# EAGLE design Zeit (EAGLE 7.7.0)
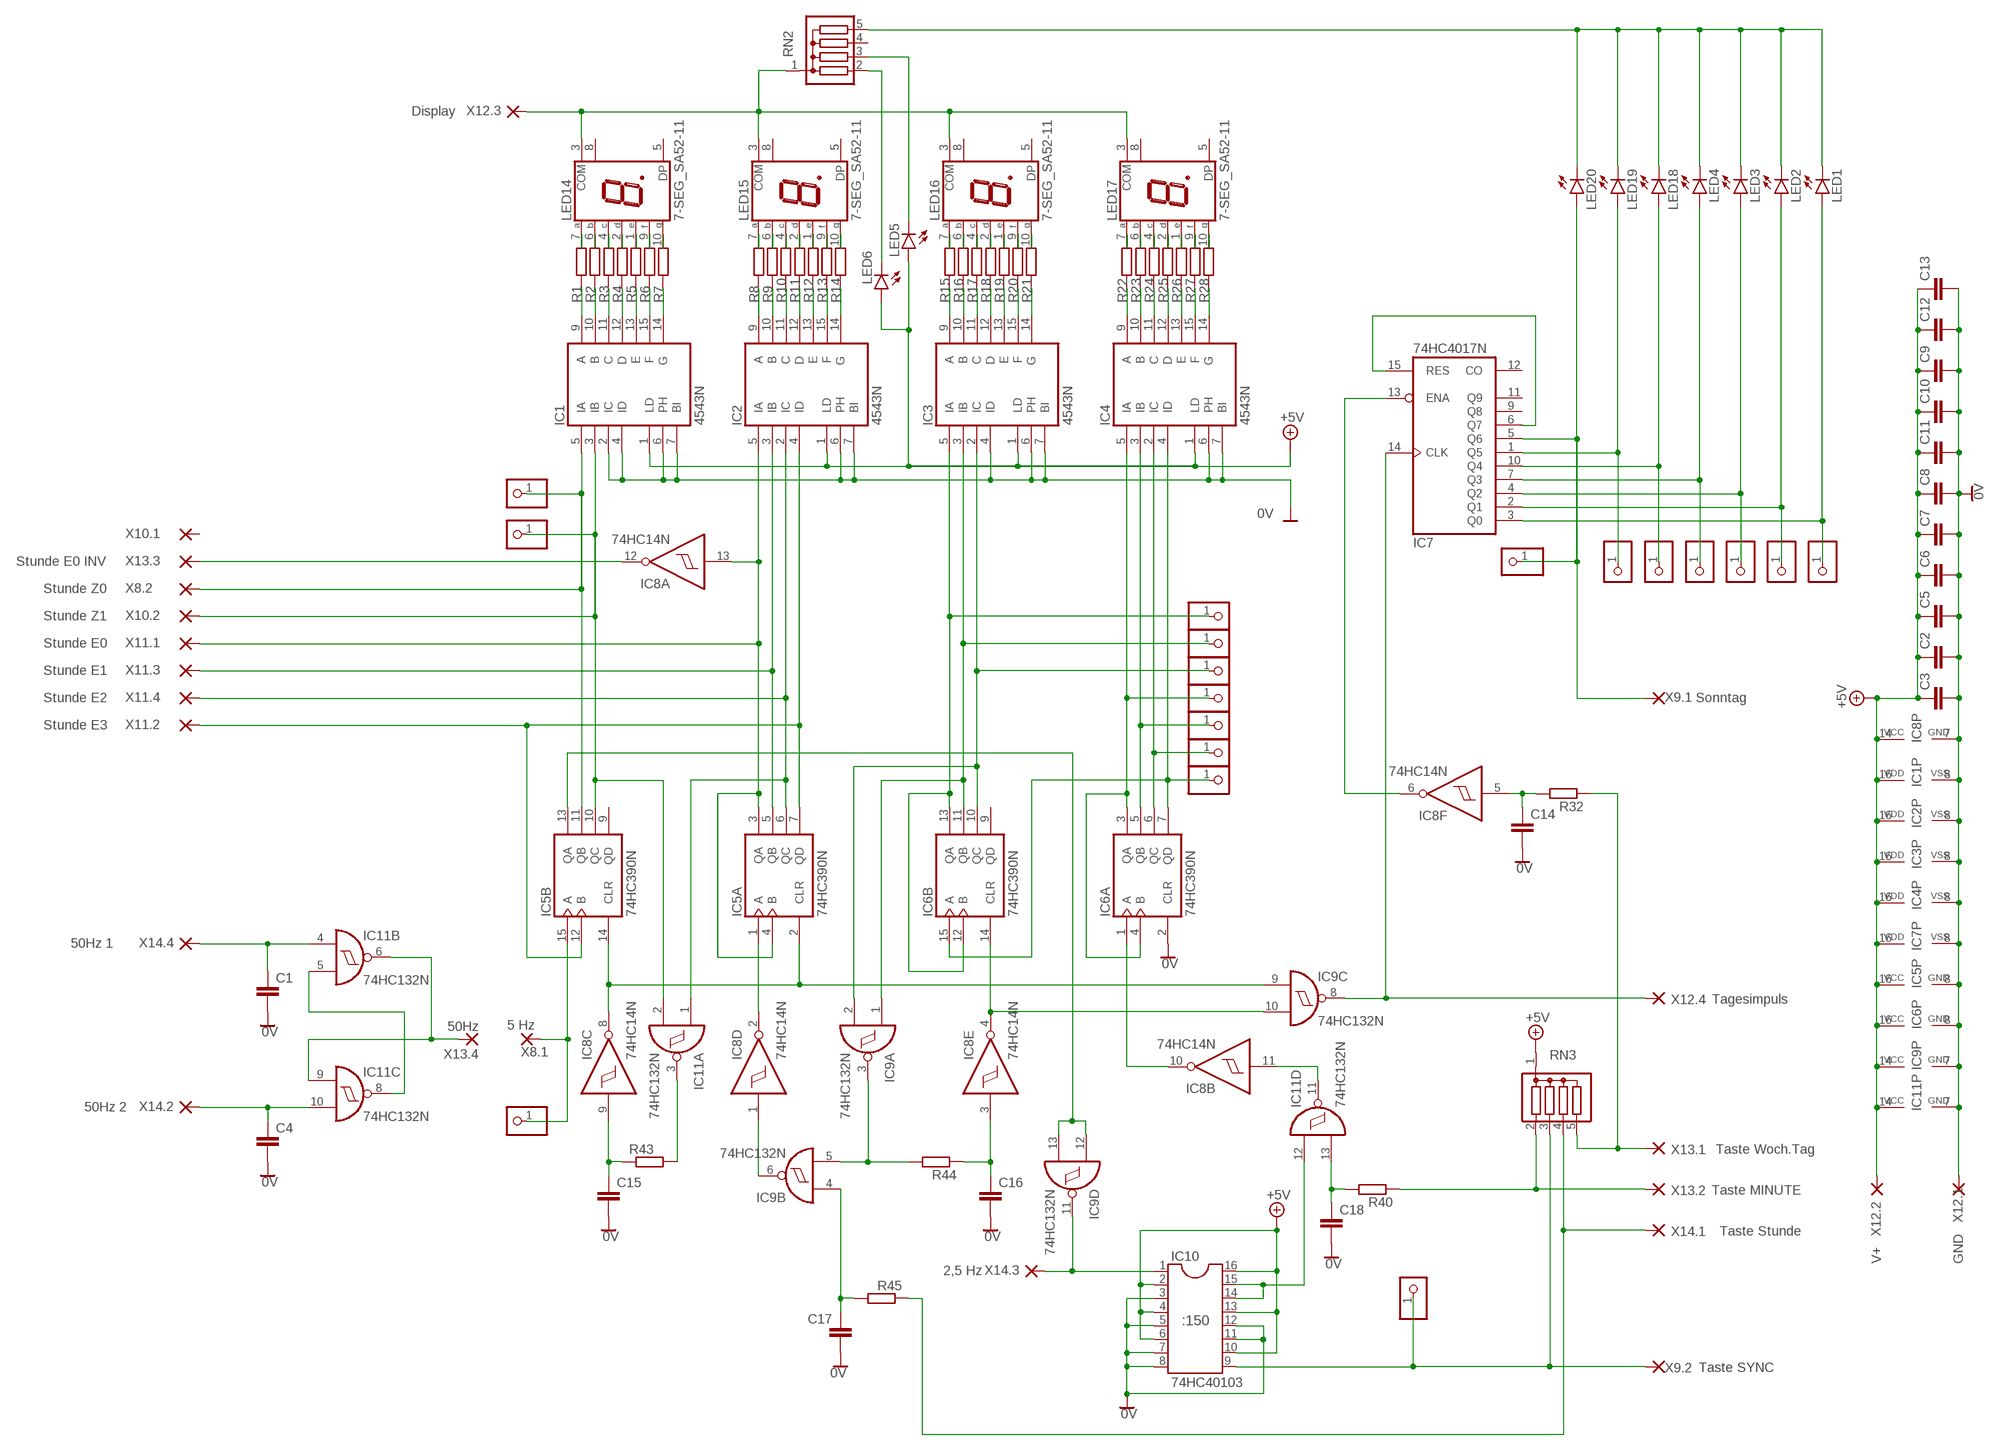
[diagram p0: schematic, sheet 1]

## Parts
101  STD Z0  PINHD-1X1  [1X01]
102  STD Z1  PINHD-1X1  [1X01]
103  MIN Z0  PINHD-1X1  [1X01]
106  MIN Z2  PINHD-1X1  [1X01]
107  MIN E2  PINHD-1X1  [1X01]
108  MIN E3  PINHD-1X1  [1X01]
109  5HZ IN  PINHD-1X1  [1X01]
110  MIN E0  PINHD-1X1  [1X01]
111  MIN Z1  PINHD-1X1  [1X01]
113  T_SYNC  PINHD-1X1  [1X01]
114  MIN E1  PINHD-1X1  [1X01]
123  PINHD-1X1  [1X01]
124  PINHD-1X1  [1X01]
125  PINHD-1X1  [1X01]
126  PINHD-1X1  [1X01]
127  PINHD-1X1  [1X01]
130  PINHD-1X1  [1X01]
133  SON  PINHD-1X1  [1X01]
C1  C-EU050-024X044  [C050-024X044]
C2  C-EU050-024X044  [C050-024X044]
C3  C-EU050-024X044  [C050-024X044]
C4  C-EU050-024X044  [C050-024X044]
C5  C-EU050-024X044  [C050-024X044]
C6  C-EU050-024X044  [C050-024X044]
C7  C-EU050-024X044  [C050-024X044]
C8  C-EU050-024X044  [C050-024X044]
C9  C-EU050-024X044  [C050-024X044]
C10  C-EU050-024X044  [C050-024X044]
C11  C-EU050-024X044  [C050-024X044]
C12  C-EU050-024X044  [C050-024X044]
C13  C-EU050-024X044  [C050-024X044]
C14  C-EU050-024X044  [C050-024X044]
C15  C-EU050-024X044  [C050-024X044]
C16  C-EU050-024X044  [C050-024X044]
C17  C-EU050-024X044  [C050-024X044]
C18  C-EU050-024X044  [C050-024X044]
IC1  4543N  [DIL16]
IC2  4543N  [DIL16]
IC3  4543N  [DIL16]
IC4  4543N  [DIL16]
IC5  74HC390N  [DIL16]
IC6  74HC390N  [DIL16]
IC7  74HC4017N  4017N  [DIL16]
IC8  74HC14N  [DIL14]
IC9  74HC132N  [DIL14]
IC10  74HC40103  DIL16  [DIL16]
IC11  74HC132N  [DIL14]
LED1  LEDSQR2X5  [LED2X5]
LED2  LEDSQR2X5  [LED2X5]
LED3  LEDSQR2X5  [LED2X5]
LED4  LEDSQR2X5  [LED2X5]
LED5  LEDSQR2X5  [LED2X5]
LED6  LEDSQR2X5  [LED2X5]
LED14  7-SEG_SA52-11  [SA52-11]
LED15  7-SEG_SA52-11  [SA52-11]
LED16  7-SEG_SA52-11  [SA52-11]
LED17  7-SEG_SA52-11  [SA52-11]
LED18  LEDSQR2X5  [LED2X5]
LED19  LEDSQR2X5  [LED2X5]
LED20  LEDSQR2X5  [LED2X5]
R1  R-EU_0207/2V  [0207/2V]
R2  R-EU_0207/2V  [0207/2V]
R3  R-EU_0207/2V  [0207/2V]
R4  R-EU_0207/2V  [0207/2V]
R5  R-EU_0207/2V  [0207/2V]
R6  R-EU_0207/2V  [0207/2V]
R7  R-EU_0207/2V  [0207/2V]
R8  R-EU_0207/2V  [0207/2V]
R9  R-EU_0207/2V  [0207/2V]
R10  R-EU_0207/2V  [0207/2V]
R11  R-EU_0207/2V  [0207/2V]
R12  R-EU_0207/2V  [0207/2V]
R13  R-EU_0207/2V  [0207/2V]
R14  R-EU_0207/2V  [0207/2V]
R15  R-EU_0207/2V  [0207/2V]
R16  R-EU_0207/2V  [0207/2V]
R17  R-EU_0207/2V  [0207/2V]
R18  R-EU_0207/2V  [0207/2V]
R19  R-EU_0207/2V  [0207/2V]
R20  R-EU_0207/2V  [0207/2V]
R21  R-EU_0207/2V  [0207/2V]
R22  R-EU_0207/2V  [0207/2V]
R23  R-EU_0207/2V  [0207/2V]
R24  R-EU_0207/2V  [0207/2V]
R25  R-EU_0207/2V  [0207/2V]
R26  R-EU_0207/2V  [0207/2V]
R27  R-EU_0207/2V  [0207/2V]
R28  R-EU_0207/2V  [0207/2V]
R32  R-EU_0207/2V  [0207/2V]
R40  R-EU_0207/2V  [0207/2V]
R43  R-EU_0207/2V  [0207/2V]
R44  R-EU_0207/2V  [0207/2V]
R45  R-EU_0207/2V  [0207/2V]
RN2  G04R  [SIL5]
RN3  G04R  [SIL5]
X8.1  5 Hz  WIREPAD1,6/0,8  [1,6/0,8]
X8.2  Stunde Z0  WIREPAD1,6/0,8  [1,6/0,8]
X9.1  Sonntag  WIREPAD1,6/0,8  [1,6/0,8]
X9.2  Taste SYNC  WIREPAD1,6/0,8  [1,6/0,8]
X10.1  WIREPAD1,6/0,8  [1,6/0,8]
X10.2  Stunde Z1  WIREPAD1,6/0,8  [1,6/0,8]
X11.1  Stunde E0  WIREPAD1,6/0,8  [1,6/0,8]
X11.2  Stunde E3  WIREPAD1,6/0,8  [1,6/0,8]
X11.3  Stunde E1  WIREPAD1,6/0,8  [1,6/0,8]
X11.4  Stunde E2  WIREPAD1,6/0,8  [1,6/0,8]
X12.1  GND  WIREPAD1,6/0,8  [1,6/0,8]
X12.2  V+  WIREPAD1,6/0,8  [1,6/0,8]
X12.3  Display  WIREPAD1,6/0,8  [1,6/0,8]
X12.4  Tagesimpuls  WIREPAD1,6/0,8  [1,6/0,8]
X13.1  Taste Woch.Tag  WIREPAD1,6/0,8  [1,6/0,8]
X13.2  Taste MINUTE  WIREPAD1,6/0,8  [1,6/0,8]
X13.3  Stunde E0 INV  WIREPAD1,6/0,8  [1,6/0,8]
X13.4  50Hz  WIREPAD1,6/0,8  [1,6/0,8]
X14.1  Taste Stunde  WIREPAD1,6/0,8  [1,6/0,8]
X14.2  50Hz 2  WIREPAD1,6/0,8  [1,6/0,8]
X14.3  2,5 Hz  WIREPAD1,6/0,8  [1,6/0,8]
X14.4  50Hz 1  WIREPAD1,6/0,8  [1,6/0,8]

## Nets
0V: C1.2 C2.2 C3.2 C4.2 C5.2 C6.2 C7.2 C8.2 C9.2 C10.2 C11.2 C12.2 C13.2 C14.2 C15.2 C16.2 C17.2 C18.2 IC1.2(IC) IC1.4(ID) IC1.6(PH) IC1.7(BI) IC1.8(VSS) IC2.6(PH) IC2.7(BI) IC2.8(VSS) IC3.4(ID) IC3.6(PH) IC3.7(BI) IC3.8(VSS) IC4.6(PH) IC4.7(BI) IC4.8(VSS) IC5.8(P:GND) IC6.2(A:CLR) IC6.8(P:GND) IC7.8(VSS) IC8.7(P:GND) IC9.7(P:GND) IC10.3 IC10.5 IC10.7 IC10.8 IC10.11 IC10.12 IC11.7(P:GND) X12.1.1(P)
+5V: C2.1 C3.1 C5.1 C6.1 C7.1 C8.1 C9.1 C10.1 C11.1 C12.1 C13.1 IC1.1(LD) IC1.16(VDD) IC2.1(LD) IC2.16(VDD) IC3.1(LD) IC3.16(VDD) IC4.1(LD) IC4.16(VDD) IC5.16(P:VCC) IC6.16(P:VCC) IC7.16(VDD) IC8.14(P:VCC) IC9.14(P:VCC) IC10.2 IC10.4 IC10.6 IC10.10 IC10.13 IC10.16 IC11.14(P:VCC) LED5.A LED6.A RN3.1 X12.2.1(P)
N$1: LED17.7(A) R22.2
N$2: LED17.6(B) R23.2
N$3: LED17.4(C) R24.2
N$4: LED17.2(D) R25.2
N$5: LED17.1(E) R26.2
N$6: LED17.9(F) R27.2
N$7: LED17.10(G) R28.2
N$8: LED16.7(A) R15.2
N$9: LED16.6(B) R16.2
N$10: LED16.4(C) R17.2
N$11: LED16.2(D) R18.2
N$12: LED16.1(E) R19.2
N$13: LED16.9(F) R20.2
N$14: LED16.10(G) R21.2
N$15: LED15.7(A) R8.2
N$16: LED15.6(B) R9.2
N$17: LED15.4(C) R10.2
N$18: LED15.2(D) R11.2
N$19: LED15.1(E) R12.2
N$20: LED15.9(F) R13.2
N$21: LED15.10(G) R14.2
N$22: LED14.7(A) R1.2
N$23: LED14.6(B) R2.2
N$24: LED14.4(C) R3.2
N$25: LED14.2(D) R4.2
N$26: LED14.1(E) R5.2
N$27: LED14.9(F) R6.2
N$28: LED14.10(G) R7.2
N$29: IC1.9(A) R1.1
N$30: IC1.10(B) R2.1
N$31: IC1.11(C) R3.1
N$32: IC1.12(D) R4.1
N$33: IC1.13(E) R5.1
N$34: IC1.15(F) R6.1
N$35: IC1.14(G) R7.1
N$36: IC2.9(A) R8.1
N$37: IC2.10(B) R9.1
N$38: IC2.11(C) R10.1
N$39: IC2.12(D) R11.1
N$40: IC2.13(E) R12.1
N$41: IC2.15(F) R13.1
N$42: IC2.14(G) R14.1
N$43: IC3.9(A) R15.1
N$44: IC3.10(B) R16.1
N$45: IC3.11(C) R17.1
N$46: IC3.12(D) R18.1
N$47: IC3.13(E) R19.1
N$48: IC3.15(F) R20.1
N$49: IC3.14(G) R21.1
N$50: IC4.9(A) R22.1
N$51: IC4.10(B) R23.1
N$52: IC4.11(C) R24.1
N$53: IC4.12(D) R25.1
N$54: IC4.13(E) R26.1
N$55: IC4.15(F) R27.1
N$56: IC4.14(G) R28.1
N$57: 111.1 IC3.3(IB) IC6.11(B:QB) IC9.1(A:I0)
N$58: IC8.12(A:O) X13.3.1(P)
N$59: 102.1 IC1.3(IB) IC5.10(B:QC) IC11.2(A:I1) X10.2.1(P)
N$60: 101.1 IC1.5(IA) IC5.11(B:QB) X8.2.1(P)
N$61: IC2.5(IA) IC5.3(A:QA) IC5.4(A:B) IC8.13(A:I) X11.1.1(P)
N$62: IC2.3(IB) IC5.5(A:QB) X11.3.1(P)
N$63: IC2.2(IC) IC5.6(A:QC) IC11.1(A:I0) X11.4.1(P)
N$64: IC2.4(ID) IC5.7(A:QD) IC5.12(B:B) X11.2.1(P)
N$65: 103.1 IC3.5(IA) IC6.12(B:B) IC6.13(B:QA)
N$66: IC6.14(B:CLR) IC8.4(E:O) IC9.10(C:I1)
N$67: IC5.1(A:A) IC8.2(D:O)
N$68: IC5.2(A:CLR) IC5.14(B:CLR) IC8.8(C:O) IC9.9(C:I0)
N$69: IC7.14(CLK) IC9.8(C:O) X12.4.1(P)
N$70: 114.1 IC4.3(IB) IC6.5(A:QB)
N$71: 107.1 IC4.2(IC) IC6.6(A:QC)
N$72: 108.1 IC4.4(ID) IC6.7(A:QD) IC6.15(B:A)
N$73: IC6.1(A:A) IC8.10(B:O)
N$74: 125.1 IC7.2(Q1) LED2.A
N$75: 126.1 IC7.4(Q2) LED3.A
N$76: 124.1 IC7.7(Q3) LED4.A
N$77: 127.1 IC7.10(Q4) LED18.A
N$78: 130.1 IC7.1(Q5) LED19.A
N$79: 133.1 IC7.5(Q6) LED20.A X9.1.1(P)
N$80: IC7.6(Q7) IC7.15(RES)
N$81: LED1.K(C) LED2.K(C) LED3.K(C) LED4.K(C) LED18.K(C) LED19.K(C) LED20.K(C) RN2.5
N$82: 106.1 IC3.2(IC) IC6.10(B:QC) IC9.2(A:I1)
N$84: LED5.K(C) RN2.3
N$85: LED6.K(C) RN2.2
N$86: 109.1 IC5.15(B:A) X8.1.1(P)
N$87: IC7.13(ENA) IC8.6(F:O)
N$88: C14.1 IC8.5(F:I) R32.2
N$89: R32.1 RN3.5 X13.1.1(P)
N$90: IC11.6(B:O) IC11.9(C:I0) X13.4.1(P)
N$91: 123.1 IC7.3(Q0) LED1.A
N$92: LED14.3(COM) LED15.3(COM) LED16.3(COM) LED17.3(COM) RN2.1 X12.3.1(P)
N$93: IC11.5(B:I1) IC11.8(C:O)
N$94: C1.1 IC11.4(B:I0) X14.4.1(P)
N$96: C4.1 IC11.10(C:I1) X14.2.1(P)
N$98: IC5.13(B:QA) IC9.12(D:I0) IC9.13(D:I1)
N$99: R45.1 RN3.4 X14.1.1(P)
N$100: IC10.14 IC10.15 IC11.12(D:I0)
N$101: IC8.11(B:I) IC11.11(D:O)
N$106: IC9.11(D:O) IC10.1 X14.3.1(P)
N$107: 110.1 IC4.5(IA) IC6.3(A:QA) IC6.4(A:B)
N$108: 113.1 IC10.9 RN3.3 X9.2.1(P)
N$109: C18.1 IC11.13(D:I1) R40.2
N$110: R40.1 RN3.2 X13.2.1(P)
N$111: C17.1 IC9.4(B:I0) R45.2
N$112: IC11.3(A:O) R43.2
N$113: C15.1 IC8.9(C:I) R43.1
N$114: IC9.3(A:O) IC9.5(B:I1) R44.2
N$115: C16.1 IC8.3(E:I) R44.1
N$116: IC8.1(D:I) IC9.6(B:O)
Unconnected: IC5.9(B:QD) IC6.9(B:QD) IC7.9(Q8) IC7.11(Q9) IC7.12(CO) LED14.5(DP) LED14.8(COM) LED15.5(DP) LED15.8(COM) LED16.5(DP) LED16.8(COM) LED17.5(DP) LED17.8(COM) RN2.4 X10.1.1(P)

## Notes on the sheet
- :150

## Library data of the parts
101-103 106-111 113 114 123-127 130 133 = pinheadxrund:PINHD-1X1: PIN HEADER
C1-C18 = rclxrund:C-EU: CAPACITOR, European symbol; SPICEPREFIX: C
IC1-IC4 = 45xxrund:4543: BCD to 7-segment LCD DECODER
IC5 IC6 = 74xx-eu:74*390: Dual 4-bit decade and binary COUNTER
IC7 = 40xxrund:4017: COUNTER/DIVIDER
IC8 = 74xx-eu:74*14: Hex schmitt trigger INVERTER
IC9 IC11 = 74xx-eu:74*132: Quad 2-input NAND schmitt trigger
IC10 = ic-packagexrund:DIL16: Dual In Line / Socket
LED1-LED6 LED18-LED20 = ledxrund:LED: LED
LED14-LED17 = display-kingbrightyx:7-SEG_: Kingbright 14.2mm (0.56 INCH) SINGLE DIGIT NUMERIC DUISPLAY Source: SA56-11EWA(Ver1189471036.pdf; OC_FARNELL: unknown; OC_NEWARK: unknown
R1-R28 R32 R40 R43-R45 = rclxrund:R-EU_: RESISTOR, European symbol; SPICEPREFIX: R
RN2 RN3 = resistor-silxrund:G04R: SIL RESISTOR; OC_FARNELL: unknown; OC_NEWARK: unknown
X8.1 X8.2 X9.1 X9.2 X10.1 X10.2 X11.1-X11.4 X12.1-X12.4 X13.1-X13.4 X14.1-X14.4 = wirepad:WIREPAD: Wire PAD connect wire on PCB

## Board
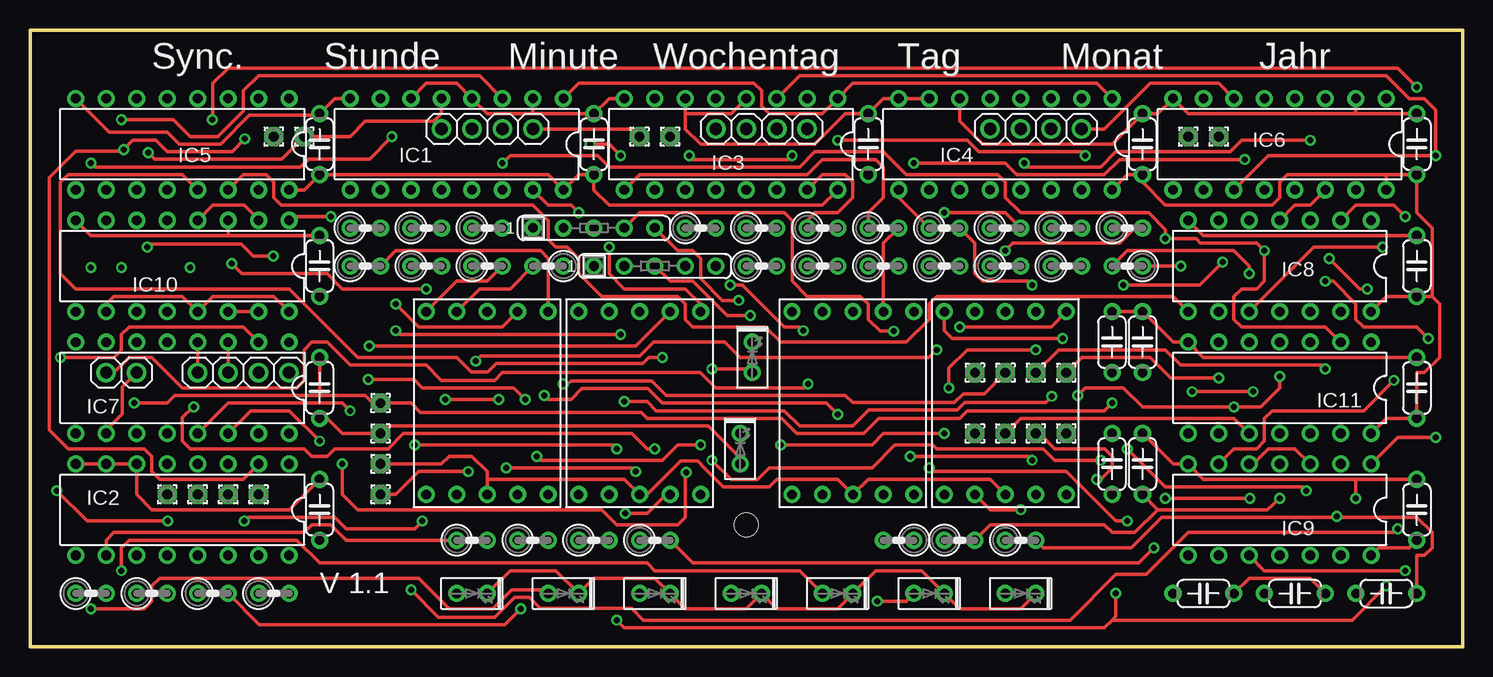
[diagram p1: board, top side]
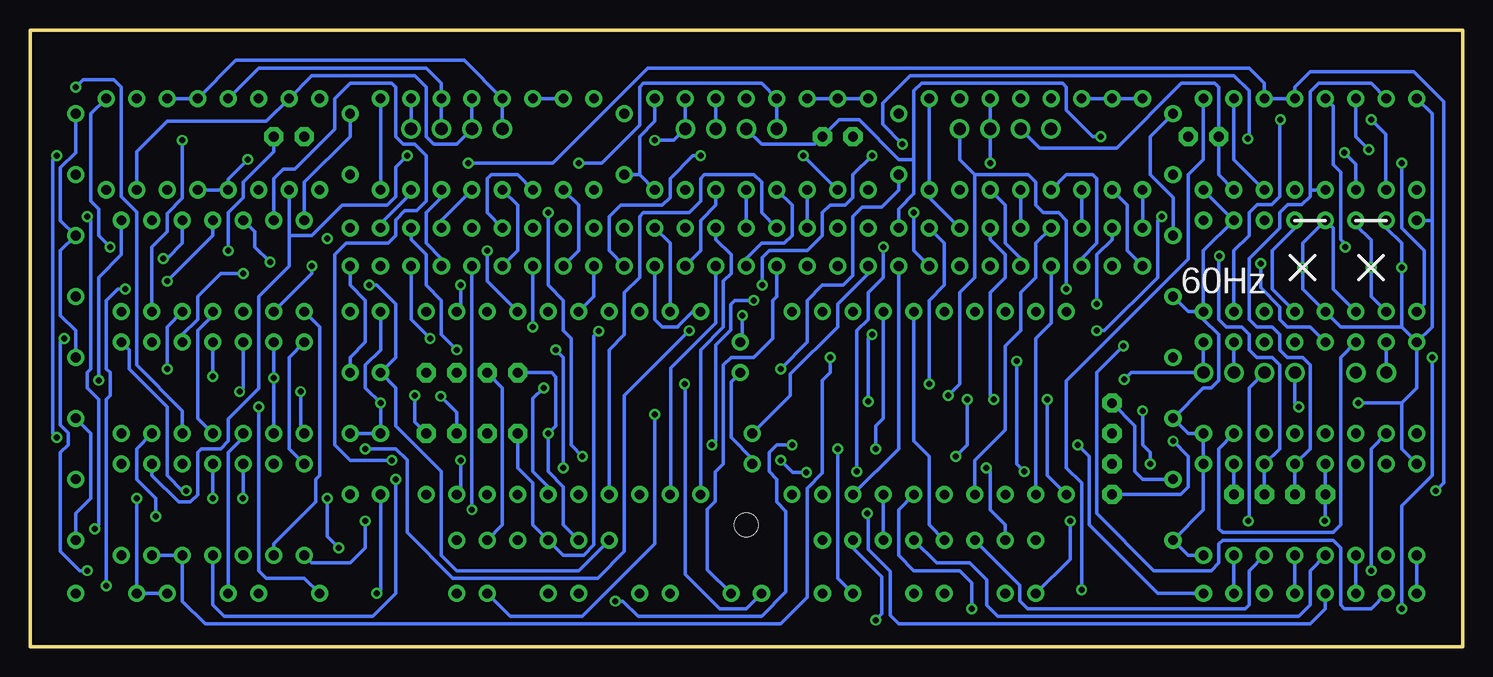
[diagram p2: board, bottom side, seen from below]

Size 119.38 x 51.44 mm. Coordinates in mm from the lower left corner, seen from the top.
Outline: 0,51.44 119.38,51.44 119.38,0 0,0 0,51.44
Copper layers (1*16): Top 0.035mm / dielectric 1.5mm / Bottom 0.035mm
Design rules "12mil *": minimum track width 12mil, minimum drill 0.5mm, track to track 12mil, track to pad 14mil, pad to pad 12mil, via to via 12mil, smd to smd 6mil, copper to edge 40mil, drill to drill 12mil, minimum pad ring 12mil, minimum via ring 8mil, stop-mask expansion 4mil, vias tented up to drill 0mil, thermal gap 10mil
Holes 2 mm at 59.69,10.16

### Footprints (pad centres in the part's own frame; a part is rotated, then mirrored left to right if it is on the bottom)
1X01 = drill 1.016: 1 0,0
C050-024X044 = drill 0.813: 1 -2.54,0; 2 2.54,0
DIL16 = drill 0.813: 1 -8.89,-3.81; 2 -6.35,-3.81; 3 -3.81,-3.81; 4 -1.27,-3.81; 5 1.27,-3.81; 6 3.81,-3.81; 7 6.35,-3.81; 8 8.89,-3.81; 9 8.89,3.81; 10 6.35,3.81; 11 3.81,3.81; 12 1.27,3.81; 13 -1.27,3.81; 14 -3.81,3.81; 15 -6.35,3.81; 16 -8.89,3.81
DIL14 = drill 0.813: 1 -7.62,-3.81; 2 -5.08,-3.81; 3 -2.54,-3.81; 4 0,-3.81; 5 2.54,-3.81; 6 5.08,-3.81; 7 7.62,-3.81; 8 7.62,3.81; 9 5.08,3.81; 10 2.54,3.81; 11 0,3.81; 12 -2.54,3.81; 13 -5.08,3.81; 14 -7.62,3.81
LED2X5 = drill 0.813: A -1.27,0; K 1.27,0
SA52-11 = drill 0.8: 1 -5.08,-7.62; 2 -2.54,-7.62; 3 0,-7.62; 4 2.54,-7.62; 5 5.08,-7.62; 6 5.08,7.62; 7 2.54,7.62; 8 0,7.62; 9 -2.54,7.62; 10 -5.08,7.62
0207/2V = drill 0.813: 1 -1.27,0; 2 1.27,0
SIL5 = drill 0.813: 1 -5.08,0; 2 -2.54,0; 3 0,0; 4 2.54,0; 5 5.08,0
1,6/0,8 = drill 0.813 pad 1.6 octagon: 1 0,0

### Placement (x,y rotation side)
101  34.29,43.18 0 top
102  39.37,43.18 0 top
103  57.15,43.18 0 top
106  64.77,43.18 0 top
107  87.63,43.18 0 top
108  82.55,43.18 0 top
109  36.83,43.18 0 top
110  80.01,43.18 0 top
111  62.23,43.18 0 top
113  59.69,43.18 0 top
114  85.09,43.18 0 top
123  16.51,22.86 0 top
124  6.35,22.86 0 top
125  19.05,22.86 0 top
126  13.97,22.86 0 top
127  8.89,22.86 0 top
130  21.59,22.86 0 top
133  41.91,43.18 0 top
C1  97.79,4.45 0 top
C2  24.13,21.59 90 top
C3  24.13,31.75 90 top
C4  105.41,4.45 0 top
C5  46.99,41.91 90 top
C6  69.85,41.91 90 top
C7  92.71,41.91 90 top
C8  115.57,11.43 90 top
C9  115.57,41.91 90 top
C10  24.13,11.43 90 top
C11  115.57,21.59 90 top
C12  115.57,31.75 90 top
C13  24.13,41.91 90 top
C14  90.17,25.4 90 top
C15  92.71,25.4 90 top
C16  90.17,15.24 90 top
C17  92.71,15.24 90 top
C18  113.03,4.45 180 top
IC1  35.56,41.91 180 top
IC2  12.7,11.43 180 top
IC3  58.42,41.91 180 top
IC4  81.28,41.91 180 top
IC5  12.7,41.91 180 top
IC6  104.14,41.91 180 top
IC7  12.7,21.59 180 top
IC8  104.14,31.75 180 top
IC9  104.14,11.43 180 top
IC10  12.7,31.75 180 top
IC11  104.14,21.59 180 top
LED1  36.83,4.45 0 top
LED2  44.45,4.45 0 top
LED3  52.07,4.45 0 top
LED4  59.69,4.45 0 top
LED5  60.2,24.13 90 top
LED6  59.18,16.51 90 top
LED14  38.1,20.32 0 top
LED15  50.8,20.32 0 top
LED16  68.58,20.32 0 top
LED17  81.28,20.32 0 top
LED18  67.31,4.45 0 top
LED19  74.93,4.45 0 top
LED20  82.55,4.45 0 top
R1  27.94,34.92 0 top
R2  27.94,31.75 0 top
R3  33.02,34.92 0 top
R4  33.02,31.75 0 top
R5  38.1,34.92 0 top
R6  43.18,31.75 180 top
R7  38.1,31.75 0 top
R8  5.08,4.45 0 top
R9  36.83,8.89 0 top
R10  10.16,4.45 0 top
R11  46.99,8.89 0 top
R12  15.24,4.45 0 top
R13  20.32,4.45 0 top
R14  41.91,8.89 0 top
R15  71.12,34.92 0 top
R16  71.12,31.75 0 top
R17  55.88,34.92 0 top
R18  60.96,31.75 0 top
R19  60.96,34.92 0 top
R20  66.04,34.92 0 top
R21  66.04,31.75 0 top
R22  76.2,34.92 0 top
R23  76.2,31.75 0 top
R24  81.28,34.92 0 top
R25  81.28,31.75 0 top
R26  86.36,34.92 0 top
R27  91.44,34.92 0 top
R28  86.36,31.75 0 top
R32  72.39,8.89 180 top
R40  82.55,8.89 0 top
R43  91.44,31.75 180 top
R44  52.07,8.89 0 top
R45  77.47,8.89 0 top
RN2  52.07,31.75 0 top
RN3  46.99,34.92 0 top
X8.1  20.32,42.55 0 top
X8.2  22.86,42.55 0 top
X9.1  50.8,42.55 0 top
X9.2  53.34,42.55 0 top
X10.1  96.52,42.55 0 top
X10.2  99.06,42.55 0 top
X11.1  11.43,12.7 0 top
X11.2  13.97,12.7 0 top
X11.3  16.51,12.7 0 top
X11.4  19.05,12.7 0 top
X12.1  29.21,20.32 0 top
X12.2  29.21,17.78 0 top
X12.3  29.21,15.24 0 top
X12.4  29.21,12.7 0 top
X13.1  78.74,22.86 0 top
X13.2  81.28,22.86 0 top
X13.3  83.82,22.86 0 top
X13.4  86.36,22.86 0 top
X14.1  78.74,17.78 0 top
X14.2  81.28,17.78 0 top
X14.3  83.82,17.78 0 top
X14.4  86.36,17.78 0 top

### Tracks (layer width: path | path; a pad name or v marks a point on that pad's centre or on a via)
0V  (via drill 0.5)
  Top 0.305: C3.2 16.51,34.29 | 16.51,34.29 5.08,34.29 IC10.8 | C2.2 24.13,20.95 | 24.13,20.95 12.06,20.95 11.43,20.32 v8.68,20.32 | C10.2 21.59,11.43 10.16,11.43 8.89,12.7 IC2.6 IC2.7 IC2.8 | 41.91,44.45 C5.2 48.26,45.72 IC3.8 | 54.61,44.45 54.61,43.18 55.88,41.91 65.41,41.91 67.94,44.45 C6.2 71.12,45.72 IC4.8 IC4.7 | 54.61,44.45 IC3.6 | IC4.6 77.47,43.81 79.38,41.91 90.17,41.91 C7.2 93.98,44.45 IC6.8 96.52,44.45 110.49,44.45 | C9.2 110.49,44.45 | C12.2 97.79,34.29 IC8.7 | C11.2 97.79,24.13 IC11.7 95.25,25.4 C15.2 C14.2 | C8.2 110.49,13.97 | 110.49,13.97 97.79,13.97 IC9.7 95.25,15.24 C17.2 | C1.2 101.6,5.71 106.68,5.71 C4.2 | 110.49,13.97 v110.49,12.38 | 24.13,20.95 27.94,20.95 28.57,20.32 X12.1.1 31.75,20.32 32.53,19.54 50.95,19.54 51.44,19.05 62.64,19.05 63.88,17.8 69.47,17.8 70.71,19.05 77.47,19.05 78.11,19.68 89.53,19.68 v90.17,20.32 | 16.51,34.29 IC10.3 | IC1.6 33.02,46.99 35.56,46.99 IC1.4 38.1,44.45 41.91,44.45 | IC3.4 58.42,44.45 54.61,44.45 | 110.49,44.45 IC6.2 | IC1.8 25.4,45.72 C13.2 24,44.32 18.29,44.32 15.88,41.91 12.45,41.91 11.43,42.93 6.6,42.93 IC5.8 | 41.91,44.45 IC1.2
  Bottom 0.305: C4.2 C18.2 v110.49,12.38 | C17.2 C16.2 v90.17,20.32 91.44,21.59 91.44,23.5 90.17,24.77 C14.2 | IC11.7 97.79,24.13 97.79,16.51 IC9.7 | C11.2 115.57,26.35 116.84,27.62 116.84,33.02 C12.2 116.84,35.56 116.84,39.94 115.57,41.21 C9.2 | C10.2 26.67,13.97 27.3,14.61 27.3,18.41 X12.1.1 | 2.54,35.56 IC10.8 | 2.54,35.56 2.54,44.45 IC5.8 | IC1.8 IC1.7 IC1.6 | IC3.8 IC3.7 IC3.6 | IC4.6 IC4.7 | IC7.8 2.54,26.67 2.54,35.56 | IC10.11 10.79,29.84 10.79,34.92 IC10.5 13.34,33.66 v13.34,31.62 13.34,29.84 IC10.12 10.16,26.67 5.08,26.67 | IC7.8 3.81,21.59 5.08,20.32 | 5.08,20.32 v8.68,20.32 | IC2.8 5.08,16.51 5.08,20.32 | C13.2 26.04,42.55 26.04,39.37 24.13,37.47 C3.2 | IC8.7 96.52,38.73 92.71,42.55 C7.2 | IC7.8 5.08,26.67 | IC10.7 6.35,34.92 5.08,33.66 v5.08,31.62 5.08,26.67
+5V  (via drill 0.5)
  Top 0.305: IC4.16 91.44,39.37 C7.1 92.71,38.73 94.61,36.83 103.5,36.83 104.14,37.47 104.14,38.73 104.78,39.37 113.03,39.37 | IC4.1 88.9,46.99 68.58,46.99 IC3.1 66.04,44.45 61.59,44.45 60.96,45.09 60.96,46.35 60.33,46.99 45.72,46.99 IC1.1 | IC9.14 112.39,8.26 114.94,8.26 C8.1 | IC11.14 113.03,19.05 C11.1 115.57,22.86 116.2,22.86 117.47,24.13 117.47,28.57 116.84,29.21 | IC8.14 113.03,29.21 C12.1 116.84,29.21 | 116.84,29.21 116.84,34.92 115.57,36.2 C9.1 113.03,39.37 | v56.83,23.18 59.69,23.18 60.01,22.86 LED5.A | C2.1 24.77,19.05 26.04,17.78 X12.2.1 29.84,18.41 56.52,18.41 59.18,15.75 LED6.A | IC5.16 22.86,38.1 C13.1 43.18,39.37 IC1.16 45.72,39.37 C5.1 46.99,38.1 48.26,36.83 66.04,36.83 IC3.16 | IC10.2 19.05,35.62 17.84,36.83 15.24,36.83 IC10.4 | IC10.16 20.32,29.21 15.24,29.21 IC10.13 12.7,29.21 6.99,29.21 6.35,28.57 IC10.10 | IC6.16 113.03,39.37
  Bottom 0.305: 68.58,39.37 68.58,42.55 67.31,43.81 IC3.1 | IC3.16 68.58,39.37 | IC4.16 IC4.1 | C8.1 115.57,11.11 114.3,12.38 114.3,17.78 C11.1 | LED6.A 59.18,15.68 60.96,17.46 60.96,22.1 LED5.A | RN3.1 44.45,37.47 IC1.16 IC1.1 | v56.83,23.18 54.61,25.4 54.61,28.89 53.34,30.16 51.6,30.16 50.8,30.96 50.8,35.88 50.01,36.67 48.42,36.67 46.99,38.1 C5.1 | IC2.16 22.86,7.62 C10.1 21.59,11.43 IC2.1 IC7.16 22.86,17.78 C2.1 21.59,21.59 20.95,21.59 20.32,22.23 20.32,26.04 21.59,27.3 IC10.16 | IC10.6 8.89,35.18 7.62,33.91 v7.62,31.62 7.62,29.21 IC10.10 | IC5.16 IC10.2 21.59,33.02 IC10.16 | 68.58,39.37 C6.1 | C3.1 22.86,27.94 IC10.16 | IC10.4 13.97,34.92 15.88,33.02 15.88,29.84 IC10.13
N$1  (via drill 0.5)
  Top 0.305: v83.5,30.16 83.19,30.48 79.38,30.48 78.74,31.11 78.74,33.66 R22.2
  Bottom 0.305: LED17.7 83.5,28.26 v83.5,30.16
N$2  (via drill 0.5)
  Top 0.305: LED17.6 85.09,26.67 v77.47,26.67
  Bottom 0.305: R23.2 v77.47,26.67
N$3  (via drill 0.5)
  Top 0.305: v83.5,15.56 83.19,15.88 v73.34,15.88 | v76.2,36.2 81.28,36.2 R24.2
  Bottom 0.305: LED17.4 83.5,13.02 v83.5,15.56 | v73.34,15.88 74.3,16.83 74.3,25.72 74.93,26.35 74.93,28.89 76.2,30.16 v76.2,36.2
N$4  (via drill 0.5)
  Top 0.305: LED17.2 80.01,11.43 v82.55,11.43
  Bottom 0.305: R25.2 v82.55,11.43
N$5  (via drill 0.5)
  Top 0.305: v83.82,24.77 78.11,24.77 76.58,23.24 v76.58,21.59
  Bottom 0.305: LED17.1 76.2,13.34 77.47,14.61 77.47,20.7 v76.58,21.59 | v83.82,24.77 85.09,26.04 85.09,28.89 86.36,30.16 86.36,32.7 87.63,33.97 R26.2
N$6  (via drill 0.5)
  Top 0.305: v81.28,33.02 81.92,33.66 90.81,33.66 92.08,34.92 R27.2
  Bottom 0.305: LED17.9 81.28,30.48 v81.28,33.02
N$7  (via drill 0.5)
  Top 0.305: v86.04,25.72 76.83,25.72 76.2,26.35 LED17.10
  Bottom 0.305: v86.04,25.72 87.63,27.3 R28.2
N$8
  Top 0.305: LED16.7 71.12,33.66 R15.2
N$9
  Bottom 0.305: LED16.6 72.39,29.21 R16.2
N$10
  Bottom 0.305: LED16.4 71.12,24.77 69.85,26.04 69.85,29.53 68.58,30.8 68.58,35.88 68.26,36.2 64.45,36.2 63.5,37.15 63.5,39.05 63.18,39.37 59.05,39.37 58.42,38.73 58.42,36.2 R17.2
N$11
  Bottom 0.305: LED16.2 65.98,12.76 65.98,23.24 62.23,26.99 R18.2
N$12
  Bottom 0.305: R19.2 62.23,33.97 60.96,32.7 60.96,31.11 61.59,30.48 61.59,26.67 63.5,24.77 LED16.1
N$13
  Bottom 0.305: LED16.9 66.04,33.66 R20.2
N$14
  Bottom 0.305: LED16.10 64.15,27.94 65.36,26.73 65.36,26.71 65.41,26.67 66.67,26.67 67.31,27.3 R21.2
N$15  (via drill 0.5)
  Top 0.305: LED15.7 50.48,25.08 v28.26,25.08
  Bottom 0.305: v28.26,25.08 30.48,22.86 30.48,11.11 25.72,6.35 20.95,6.35 20.32,6.99 20.32,8.57 20,8.89 10.79,8.89 10.16,8.26 10.16,3.49 9.84,3.17 7.62,3.17 R8.2
N$16  (via drill 0.5)
  Top 0.305: LED15.6 55.88,28.57 54.61,29.84 49.53,29.84 48.26,31.11 v48.26,33.34 | v50.48,14.61 50.16,14.92 v39.69,14.92
  Bottom 0.305: v48.26,33.34 48.26,30.8 49.53,29.53 49.53,27.3 50.48,26.35 v50.48,14.61 | v39.69,14.92 39.37,14.61 39.37,11.43 38.1,10.16 R9.2
N$17  (via drill 0.5)
  Top 0.305: v49.59,11.11 51.44,11.11 53.02,12.7 LED15.4
  Bottom 0.305: v49.59,11.11 49.53,11.05 49.53,8.13 47.69,6.29 47.69,2.6 46.99,1.91 12.7,1.91 11.43,3.17 R10.2
N$18
  Bottom 0.305: R11.2 LED15.2
N$19  (via drill 0.5)
  Top 0.305: v40.89,3.17 39.56,1.84 19.11,1.84 R12.2
  Bottom 0.305: LED15.1 46.99,11.43 46.99,7.62 45.72,6.35 41.91,6.35 40.89,5.33 v40.89,3.17
N$20  (via drill 0.5)
  Top 0.305: v48.9,16.51 48.58,16.83 v32.07,16.83
  Bottom 0.305: LED15.9 48.26,19.05 48.9,18.41 v48.9,16.51 | v32.07,16.83 31.11,15.88 31.11,10.16 25.4,4.45 R13.2
N$21
  Bottom 0.305: LED15.10 45.72,17.14 44.45,15.88 44.45,10.16 R14.2
N$22  (via drill 0.5)
  Top 0.305: LED14.7 39.37,26.67 32.38,26.67 v30.48,28.57
  Bottom 0.305: v30.48,28.57 30.48,32.7 29.21,33.97 R1.2
N$23
  Top 0.305: LED14.6 43.18,32.38 42.55,33.02 30.48,33.02 R2.2
N$24
  Bottom 0.305: LED14.4 40.64,15.56 38.1,18.1 38.1,25.08 36.83,26.35 36.83,29.53 35.56,30.8 35.56,33.66 R3.2
N$25
  Bottom 0.305: LED14.2 35.56,25.72 34.29,26.99 R4.2
N$26  (via drill 0.5)
  Top 0.305: v39.05,20.64 v34.61,20.64
  Bottom 0.305: LED14.1 34.61,14.29 v34.61,20.64 | v39.05,20.64 39.37,20.95 39.37,29.53 38.1,30.8 38.1,32.7 39.37,33.97 R5.2
N$27
  Top 0.305: LED14.9 37.47,29.84 40.01,29.84 R6.2
N$28
  Top 0.305: LED14.10 35.56,30.48 38.1,30.48 R7.2
N$29
  Bottom 0.305: IC1.9 R1.1
N$30
  Bottom 0.305: R2.1 27.94,33.02 27.94,36.83 IC1.10
N$31
  Bottom 0.305: IC1.11 R3.1
N$32
  Bottom 0.305: R4.1 31.75,32.38 30.48,33.66 30.48,39.05 30.8,39.37 33.02,39.37 IC1.12
N$33
  Bottom 0.305: IC1.13 R5.1
N$34  (via drill 0.5)
  Top 0.305: v45.72,36.2 45.09,36.83 43.18,36.83 IC1.15
  Bottom 0.305: R6.1 45.72,33.02 v45.72,36.2
N$35
  Bottom 0.305: R7.1 36.83,32.38 38.1,33.66 38.1,36.83 IC1.14
N$36
  Bottom 0.305: IC2.9 R8.1
N$37
  Top 0.305: IC2.10 6.35,8.89 6.99,9.53 22.86,9.53 23.5,10.16 25.08,10.16 26.35,8.89 R9.1
N$38
  Bottom 0.305: IC2.11 R10.1
N$39
  Bottom 0.305: IC2.12 12.7,6.35 12.7,3.49 13.65,2.54 38.73,2.54 39.65,3.45 39.65,5.59 41.05,6.99 43.81,6.99 R11.1
N$40
  Bottom 0.305: IC2.13 R12.1
N$41
  Bottom 0.305: IC2.15 R13.1
N$42
  Bottom 0.305: IC2.14 17.78,6.35 17.78,3.49 18.1,3.17 36.22,3.17 36.88,3.83 36.88,5.13 R14.1
N$43
  Top 0.305: IC3.9 50.8,39.37 64.77,39.37 66.04,40.64 70.48,40.64 71.12,40.01 71.12,37.47 69.85,36.2 R15.1
N$44  (via drill 0.5)
  Top 0.305: v63.5,40.96 63.18,40.64 55.24,40.64 v54.93,40.96
  Bottom 0.305: R16.1 71.12,33.02 71.12,35.88 70.17,36.83 66.67,36.83 66.04,37.47 66.04,39.05 64.14,40.96 v63.5,40.96 | IC3.10 v54.93,40.96
N$45
  Bottom 0.305: IC3.11 R17.1
N$46
  Bottom 0.305: R18.1 59.69,32.38 58.42,33.66 56.52,33.66 55.88,34.29 55.88,36.83 IC3.12
N$47
  Bottom 0.305: IC3.13 R19.1
N$48
  Top 0.305: IC3.15 66.04,39.37 67.94,39.37 68.58,38.73 68.58,37.47 67.31,36.2 65.41,36.2 64.77,35.56 R20.1
N$49
  Bottom 0.305: R21.1 63.5,33.02 63.5,35.56 62.23,36.83 IC3.14
N$50
  Top 0.305: R22.1 72.39,37.47 IC4.9
N$51
  Bottom 0.305: R23.1 73.66,33.02 73.66,36.83 IC4.10
N$52
  Bottom 0.305: R24.1 81.28,36.2 81.28,39.05 80.96,39.37 78.74,39.37 IC4.11
N$53
  Bottom 0.305: R25.1 78.74,33.02 78.74,36.83 IC4.12
N$54
  Bottom 0.305: IC4.13 85.09,35.56 R26.1
N$55
  Bottom 0.305: IC4.15 87.63,37.85 90.17,35.31 R27.1
N$56
  Bottom 0.305: R28.1 85.09,32.38 86.36,33.66 86.36,36.2 85.09,37.47 IC4.14
N$57  (via drill 0.5)
  Top 0.305: IC9.1 113.98,17.46 v117.16,17.46 | IC6.11 103.19,40.96 v117.16,40.96 117.16,44.77 116.2,45.72 114.94,45.72 113.03,47.62 64.14,47.62 IC3.3
  Bottom 0.305: 111.1 IC3.3 | v117.16,17.46 117.47,17.78 117.47,40.64 v117.16,40.96
N$58  (via drill 0.5)
  Top 0.305: v107.95,23.18 107.63,23.5 95.89,23.5 94.61,24.77 85.72,24.77 X13.3.1
  Bottom 0.305: IC8.12 107.95,26.67 v107.95,23.18
N$59  (via drill 0.5)
  Top 0.305: IC1.3 37.47,47.62 19.05,47.62 17.78,46.35 17.78,44.68 15.65,42.55 13.34,42.55 11.94,43.94 v7.62,43.94 | IC11.2 107.95,26.67 100.97,26.67 100.33,27.3 100.33,29.21 100.97,29.84 102.23,29.84 102.87,30.48 v102.87,33.02 102.21,33.68 97.54,33.68 97.18,34.04 v94.61,34.04 94.61,34.8 93.22,36.2 82.55,36.2 81.28,37.47 81.28,38.73 80.64,39.37 73.03,39.37 71.12,41.27 65.41,41.27 64.14,40.01 48.26,40.01 47.31,40.96 40.01,40.96 v39.37,40.32
  Bottom 0.305: v7.62,43.94 6.41,42.74 6.41,38.16 IC5.10 | v39.37,40.32 102.1 IC1.3 | v102.87,33.02 102.87,36.2 101.6,37.47 101.6,38.76 99.06,41.3 X10.2.1
N$60  (via drill 0.5)
  Top 0.305: IC1.5 34.29,44.45 33.66,43.81 | 33.66,43.81 101.1 | 33.66,43.81 27.94,43.81 26.67,42.55 X8.2.1 20.99,40.68 10.38,40.68 v9.84,41.21
  Bottom 0.305: v9.84,41.21 8.89,40.26 IC5.11
N$61  (via drill 0.5)
  Top 0.305: v106.68,42.23 100.97,42.23 100.01,41.27 90.49,41.27 89.22,40.01 83.19,40.01 v82.87,40.32 | v11.49,10.48 4.76,10.48 v2.22,13.02
  Bottom 0.305: IC2.5 X11.1.1 11.43,10.54 v11.49,10.48 | IC8.13 109.22,33.34 107.95,34.61 107.95,36.13 106.68,37.4 v106.68,42.23 | v82.87,40.32 75.82,40.32 67.88,48.26 17.78,48.26 16.51,46.99 IC5.3 IC5.4 13.97,46.67 12.7,47.94 4.06,47.94 1.59,45.47 1.59,13.65 v2.22,13.02
N$62  (via drill 0.5)
  Top 0.305: v20.26,32.58 18.61,32.58 17.59,33.59 10.03,33.59 v9.78,33.34
  Bottom 0.305: X11.3.1 IC2.3 15.24,16.51 15.24,23.5 15.88,24.13 17.14,24.13 17.78,24.77 17.78,26.04 18.41,26.67 19.68,26.67 20.32,27.3 20.32,32.51 v20.26,32.58 | IC5.5 10.79,45.09 10.79,40.2 10.16,39.56 10.16,33.97 9.78,33.59 v9.78,33.34
N$63  (via drill 0.5)
  Top 0.305: v106.36,13.02 106.05,13.34 94.61,13.34 v91.44,16.51 | v64.45,26.35 64.14,26.67 62.87,26.67 59.37,30.16 v58.36,30.16 | v49.21,40.96 48.26,41.91 v46.67,41.91 | IC2.2 17.78,13.97 10.79,13.97 10.16,14.61 10.16,15.88 9.53,16.51 3.17,16.51 1.59,18.1 1.59,39.12 3.81,41.34 7.68,41.34 v7.81,41.47 8.57,42.23 10.48,42.23 11.42,41.29 16.84,41.29 v17.91,42.35
  Bottom 0.305: X11.4.1 IC2.2 | IC11.1 111.12,24.77 111.12,23.18 107.95,20 107.95,14.29 106.68,13.02 v106.36,13.02 | v64.45,26.35 69.85,20.95 69.85,7.94 72.07,5.71 84.14,5.71 87.95,9.53 87.95,15.57 88.88,16.51 v91.44,16.51 | v46.67,41.91 48.32,43.56 48.32,45.34 46.04,47.62 19.05,47.62 17.78,46.35 17.78,42.48 v17.91,42.35 | v7.81,41.47 8.89,42.55 IC5.6 | v58.36,30.16 58.36,32.45 57.78,33.02 54.61,33.02 53.34,34.29 53.34,36.2 52.7,36.83 51.44,36.83 50.8,37.47 50.8,39.37 v49.21,40.96
N$64
  Bottom 0.305: X11.2.1 IC2.4 12.7,16.51 12.7,23.5 13.34,24.13 14.61,24.13 15.24,24.77 15.24,26.04 15.88,26.67 17.14,26.67 17.78,27.3 17.78,32.38 15.24,34.92 15.24,36.2 14.58,36.85 13.38,36.85 12.7,37.53 12.7,38.1 | 12.7,38.1 12.7,46.29 12,46.99 7.62,46.99 IC5.7 | 12.7,38.1 IC5.12
N$65  (via drill 0.5)
  Top 0.305: v73.66,40.32 81.28,40.32 82.23,39.37 89.53,39.37 90.81,40.64 v101.22,40.64
  Bottom 0.305: 103.1 IC3.5 58.42,46.99 68.26,46.99 68.58,46.67 68.58,43.5 71.75,40.32 v73.66,40.32 | v101.22,40.64 102.87,38.99 IC6.12 IC6.13
N$66  (via drill 0.5)
  Top 0.305: IC9.10 102.87,6.35 v114.62,6.35 | v116.52,25.72 115.57,26.67 111.12,26.67 110.49,27.3 110.49,28.57 108.58,30.48 v107.95,30.48 | IC6.14 106.68,36.83 105.41,36.83 IC8.4
  Bottom 0.305: v114.62,6.35 115.25,6.35 116.84,7.94 116.84,16.19 116.2,16.83 116.2,17.84 116.84,18.48 116.84,25.4 v116.52,25.72 | v107.95,30.48 104.14,34.29 IC8.4
N$67  (via drill 0.5)
  Top 0.305: v31.75,4.76 34.04,2.48 38.73,2.48 40.39,4.13 41.59,4.13 42.52,3.2 50.14,3.2 51.12,2.22 86.68,2.22 90.49,6.03 93.03,6.03 96.52,9.53 113.67,9.53 v113.98,9.84 | v114.62,35.88 113.67,36.83 110.49,36.83 IC8.2
  Bottom 0.305: v31.75,4.76 31.75,13.65 33.02,14.92 33.02,22.16 22.86,32.32 22.86,39.37 21.59,40.64 IC5.1 | v113.98,9.84 113.67,10.16 113.67,20.64 114.62,21.59 114.62,22.86 114.3,23.18 114.3,35.56 v114.62,35.88
N$68
  Top 0.305: IC8.8 95.25,29.21 75.56,29.21 74.93,28.57 74.93,27.3 73.03,25.4 62.55,25.4 61.28,26.67 55.24,26.67 54.61,27.3 54.61,28.57 53.98,29.21 47.62,29.21 45.72,31.11 45.72,32.38 44.77,33.34 43.81,33.34 43.18,33.97 43.18,35.56 41.91,36.83 20.95,36.83 20.32,37.47 20.32,38.73 19.68,39.37 17.78,39.37 IC5.14
  Bottom 0.305: IC5.14 19.05,40.64 IC5.2 | IC8.8 95.25,26.67 95.25,14.29 95.57,13.97 95.57,12.06 99.06,8.57 IC9.9
N$69  (via drill 0.5)
  Top 0.305: v91.44,10.48 90.49,10.48 86.36,14.61 75.25,14.61 v74.93,14.92 | IC7.14 18.41,19.68 21.59,19.68 v24.13,17.14 | v36.51,14.61 32.38,14.61 30.48,12.7 X12.4.1 | v37.15,23.81 37.57,24.23 50.8,24.23 51.97,25.4 57.89,25.4 59.18,24.11 74.91,24.11 v75.56,24.77
  Bottom 0.305: v74.93,14.92 74.93,24.13 v75.56,24.77 | v24.13,17.14 22.86,15.88 22.86,13.34 23.5,12.7 X12.4.1 | v36.51,14.61 37.15,15.24 v37.15,23.81 | v91.44,10.48 91.44,8.26 92.71,6.99 95.89,6.99 IC9.8
N$70
  Bottom 0.305: 114.1 IC4.3 85.09,46.99 86.36,48.26 100.33,48.26 IC6.5
N$71
  Top 0.305: IC6.6 99.06,46.99 93.34,46.99 89.53,43.18 107.1
  Bottom 0.305: 107.1 IC4.2
N$72
  Bottom 0.305: IC4.4 108.1 83.82,41.91 85.72,41.91 86.36,42.55 86.36,46.67 87.31,47.62 95.89,47.62 IC6.7 99.69,43.81 107.95,43.81 110.49,41.27 IC6.15
N$73  (via drill 0.5)
  Top 0.305: IC8.10 107,33.34 v112.71,33.34
  Bottom 0.305: v112.71,33.34 113.67,34.29 113.67,36.51 114.3,37.15 114.3,44.45 IC6.1
N$74  (via drill 0.5)
  Top 0.305: LED2.A 42.86,4.76 40.16,4.76 38.57,3.17 34.92,3.17 32.38,5.71 10.79,5.71 10.16,5.08 10.16,3.81 9.53,3.17 v5.08,3.17 | IC7.2 17.78,26.67 8.26,26.67 7.62,26.04 7.62,24.74 7.01,24.13 v2.54,24.13
  Bottom 0.305: v5.08,3.17 5.08,11.75 2.54,14.29 v2.54,24.13 | IC7.2 125.1
N$75  (via drill 0.5)
  Top 0.305: v52.07,16.51 51.44,16.51 50.16,17.78 31.11,17.78 29.84,16.51 25.4,16.51 24.77,15.88 23.5,15.88 22.86,16.51 13.34,16.51 12.7,17.14 12.7,19.11 13.59,20 v13.65,20 | 126.1 IC7.4
  Bottom 0.305: LED3.A 52.07,5.71 v52.07,16.51 | v13.65,20 13.97,20.32 126.1
N$76  (via drill 0.5)
  Top 0.305: v64.83,21.91 64.52,21.59 57.13,21.59 55.86,22.86 39.37,22.86 38.73,22.23 34.29,22.23 33.02,23.5 26.67,23.5 24.77,25.4 23.5,25.4 22.86,24.77 22.86,22.23 22.23,21.59 12.7,21.59 10.16,24.13 8.26,24.13 6.99,22.86 124.1
  Bottom 0.305: LED4.A 59.69,3.17 61.91,3.17 64.77,6.03 64.77,21.84 v64.83,21.91 | 124.1 IC7.7
N$77  (via drill 0.5)
  Top 0.305: LED18.A 64.14,6.35 52.07,6.35 51.44,6.99 24.13,6.99 22.23,8.89 8.26,8.89 7.62,8.26 v7.62,6.35 | IC7.10 6.35,18.1 7.68,19.43 7.68,21.65 127.1
  Bottom 0.305: v7.62,6.35 7.62,16.51 IC7.10
N$78  (via drill 0.5)
  Top 0.305: LED19.A 73.03,3.81 v70.61,3.81 | v55.88,16.83 53.98,16.83 52.7,15.56 42.55,15.56 v42.23,15.88 | v41.27,20.64 40.32,21.59 32.7,21.59 32,22.29 v28.19,22.29
  Bottom 0.305: IC7.1 130.1 27.62,22.86 v28.19,22.29 | v70.61,3.81 69.98,3.81 68.71,2.54 58.42,2.54 56.39,4.57 56.39,11.3 57.15,12.06 57.15,13.97 57.78,14.61 57.78,16.19 57.15,16.83 v55.88,16.83 | v42.23,15.88 41.27,16.83 v41.27,20.64
N$79  (via drill 0.5)
  Top 0.305: v67.31,19.37 66.36,20.32 52.7,20.32 51.47,21.55 46,21.55 45.09,20.64 43.18,20.64 v42.86,20.95 | v16.83,31.94 17.65,31.11 24.77,31.11 26.04,29.84 v33.02,29.84 | X9.1.1 50.16,43.18 133.1
  Bottom 0.305: LED20.A 79.38,2.54 73.34,2.54 67.31,8.57 v67.31,19.37 | v42.86,20.95 41.91,21.91 41.91,29.53 40.64,30.8 40.64,39.37 | 40.64,39.37 36.2,39.37 35.56,38.73 35.56,36.83 34.92,36.2 33.66,36.2 33.02,35.56 33.02,29.91 33.05,29.88 v33.02,29.84 | 133.1 41.91,40.64 40.64,39.37 | IC7.5 12.7,26.67 14.61,26.67 15.24,27.3 15.24,28.35 16.83,29.93 v16.83,31.94
N$80
  Bottom 0.305: IC7.15 20.32,16.51 20.32,9.84 20,9.53 10.79,9.53 10.16,10.16 10.16,24.13 IC7.6
N$81
  Top 0.305: LED1.K 40.01,6.35 43.81,6.35 LED2.K 46.99,5.71 52.07,5.71 LED3.K 54.61,3.17 59.69,3.17 LED4.K 62.23,3.17 67.31,3.17 LED18.K 70.48,6.35 74.3,6.35 LED19.K 77.47,3.17 82.55,3.17 LED20.K
  Bottom 0.305: RN2.5 57.15,29.21 57.47,28.89 57.47,25.72 59.05,24.13 60.96,24.13 61.59,23.5 61.59,15.24 62.26,14.58 62.26,12.13 62.93,11.46 62.93,6.41 LED4.K
N$82  (via drill 0.5)
  Top 0.305: v67.31,42.23 78.11,42.23 79.06,41.27 87.63,41.27 v87.95,40.96
  Bottom 0.305: IC3.2 106.1 65.72,42.23 v67.31,42.23 | IC9.2 109.22,14.29 107,12.06 106.05,12.06 106,12.11 105.98,12.11 105.41,12.68 105.41,16.19 105.09,16.51 103.5,16.51 102.87,17.14 102.87,18.99 100.33,21.53 100.33,29.21 97.79,31.75 97.79,34.29 | v87.95,40.96 88.9,40.01 88.9,37.53 89.6,36.83 93.34,36.83 95.89,34.29 97.79,34.29 | 97.79,34.29 IC6.10
N$84  (via drill 0.5)
  Top 0.305: v60.01,27.62 58.1,27.62 55.24,30.48 53.34,30.48 RN2.3
  Bottom 0.305: v60.01,27.62 60.01,25.4 LED5.K
N$85
  Bottom 0.305: LED6.K 56.01,20.95 56.01,22.73 52.07,26.67 52.07,28.57 49.53,31.11 RN2.2
N$86
  Bottom 0.305: IC5.15 20.32,39.37 X8.1.1 20.32,46.67 20.64,46.99 23.43,46.99 28.83,41.59 35.24,41.59 109.1
N$87  (via drill 0.5)
  Top 0.305: IC7.13 16.51,20.32 26.04,20.32 v26.67,19.68 | v26.04,15.24 26.04,12.7 27.3,11.43 47.62,11.43 48.9,10.16 53.98,10.16 54.61,10.79 54.61,14.48 v54.67,14.54 | v89.22,15.56 85.41,15.56 84.45,16.51 75.56,16.51 75.25,16.83 72.07,16.83 70.17,14.92 61.59,14.92 60.64,13.97 58.42,13.97 v56.83,15.56
  Bottom 0.305: v26.67,19.68 26.67,16.83 26.04,16.19 v26.04,15.24 | v54.67,14.54 55.82,14.54 v56.83,15.56 | v89.22,15.56 92.71,15.56 93.98,16.83 93.98,32.7 93.03,33.66 89.53,33.66 88.9,34.29 88.9,35.59 88.13,36.35 87.15,36.35 86.36,37.15 86.36,40.96 87.31,41.91 88.27,41.91 88.9,42.55 88.9,46.67 89.22,46.99 92.71,46.99 93.98,45.72 93.98,43.18 97.31,39.85 98.27,39.85 99.06,39.05 IC8.6
N$88  (via drill 0.5)
  Top 0.305: v99.38,32.07 97.47,30.16 v91.12,30.16
  Bottom 0.305: R32.2 73.66,6.35 83.82,6.35 85.09,7.62 85.09,14.61 88.9,18.41 88.9,21.59 C14.1 88.9,24.13 88.9,28.57 90.49,30.16 v91.12,30.16 | IC8.5 100.65,34.61 100.65,33.34 v99.38,32.07
N$89  (via drill 0.5)
  Top 0.305: RN3.5 53.98,33.02 55.24,33.02 55.88,32.38 55.88,30.71 57.7,28.89 v59.05,28.89 | v62.55,16.83 70.17,16.83 71.12,17.78 v76.2,17.78
  Bottom 0.305: R32.1 74.93,10.16 74.93,13.34 76.2,14.61 v76.2,17.78 75.56,18.41 75.56,22.51 75.92,22.86 X13.1.1 | v59.05,28.89 60.64,28.89 60.98,28.55 60.98,26.42 62.23,25.17 62.23,17.14 v62.55,16.83
N$90  (via drill 0.5)
  Top 0.305: X13.4.1 87.63,24.13 93.34,24.13 95.06,22.42 v99.06,22.42
  Bottom 0.305: IC11.6 v99.06,22.42 IC11.9
N$91  (via drill 0.5)
  Top 0.305: v32.7,10.48 32.07,9.84 26.35,9.84 25.4,10.79 18.16,10.79 v17.84,10.48 | 123.1 IC7.3
  Bottom 0.305: LED1.A 32.7,7.3 v32.7,10.48 | v17.84,10.48 17.78,10.54 17.78,21.59 123.1
N$92
  Top 0.305: LED17.3 80.01,13.97 69.85,13.97 LED16.3 67.31,13.97 62.23,13.97 61.59,13.34 57.78,13.34 57.19,13.93 57.17,13.93 55.92,15.18 55.92,15.2 55.63,15.49 54.23,15.49 51.44,12.7 LED15.3 49.53,13.97 38.1,13.97 | 38.1,13.97 38.1,14.61 36.83,15.88 34.92,15.88 34.29,15.24 X12.3.1 | 38.1,13.97 LED14.3
  Bottom 0.305: RN2.1 46.99,16.51 LED15.3
N$93  (via drill 0.5)
  Top 0.305: v101.92,21.27 v96.84,21.27
  Bottom 0.305: IC11.8 96.84,18.1 v96.84,21.27 | v101.92,21.27 101.6,21.59 IC11.5
N$94  (via drill 0.5)
  Top 0.305: v87.31,20.95 87.95,21.59 91.12,21.59 92.71,20 v100.33,20 102.55,20 104.14,21.59 v104.14,22.54
  Bottom 0.305: IC11.4 v104.14,22.54 | X14.4.1 87.31,18.73 v87.31,20.95 | C1.1 96.52,5.71 99.69,5.71 100.33,6.35 v100.33,20
N$96
  Top 0.305: X14.2.1 82.55,19.05 100.33,19.05 IC11.10
  Bottom 0.305: IC11.10 101.6,17.46 102.87,16.19 C4.1
N$98  (via drill 0.5)
  Top 0.305: IC5.13 12.7,39.37 3.17,39.37 2.54,38.73 2.54,31.11 3.81,29.84 21.59,29.84 27.3,24.13 35.54,24.13 36.77,22.9 38.14,22.9 38.86,23.62 51.05,23.62 51.56,24.13 v52.7,24.13
  Bottom 0.305: IC9.13 IC9.12 106.68,3.81 104.78,1.91 56.83,1.91 54.61,4.13 54.61,13.21 53.34,14.48 53.34,22.23 52.7,22.86 v52.7,24.13
N$99  (via drill 0.5)
  Top 0.305: RN3.4 50.8,36.2 62.87,36.2 63.5,35.56 63.5,30.48 64.77,29.21 69.21,29.21 69.85,28.57 69.85,27.3 70.84,26.31 v71.99,26.31
  Bottom 0.305: X14.1.1 78.74,14.92 77.47,13.65 77.47,10.16 R45.1 74.93,7.62 73.25,7.62 72.39,8.48 72.39,25.91 v71.99,26.31
N$100  (via drill 0.5)
  Top 0.305: v115.57,46.67 113.98,48.26 17.14,48.26 16.95,48.26 16.51,48.26 15.24,46.99 15.24,44.13 15.3,44.07 v15.18,43.94 | IC10.15 IC10.14
  Bottom 0.305: IC11.12 106.68,19.68 110.49,23.5 110.49,36.26 111.76,37.53 111.76,46.67 112.39,47.31 114.94,47.31 v115.57,46.67 | v15.18,43.94 15.24,43.88 15.24,37.53 15.91,36.85 17.12,36.85 17.78,36.2 17.78,34.29 19.05,33.02 IC10.15
N$101
  Bottom 0.305: IC11.11 105.41,19.05 105.41,26.35 104.14,27.62 IC8.11
N$106  (via drill 0.5)
  Top 0.305: v88.9,13.97 89.22,13.97 90.17,14.92 90.17,15.88 90.13,15.92 90.13,15.94 89.55,16.51 85.41,16.51 84.14,17.78 X14.3.1 | IC10.1 21.91,35.88 v25.08,35.88 | v30.48,26.35 30.8,26.04 v49.21,26.04 | v49.53,20.45 51.44,20.45 52.2,19.68 62.87,19.68 64.14,18.41 68.58,18.41 69.91,19.75 77.28,19.75 77.92,20.38 84.64,20.38 v85.15,20.89
  Bottom 0.305: IC9.11 104.14,3.49 103.19,2.54 90.81,2.54 88.9,4.45 v88.9,13.97 | v25.08,35.88 25.4,35.56 25.4,30.8 29.84,26.35 v30.48,26.35 | v49.21,26.04 49.53,25.72 v49.53,20.45 | v85.15,20.89 83.82,19.56 X14.3.1
N$107
  Bottom 0.305: IC6.3 IC6.4 102.23,48.9 83.19,48.9 IC4.5 110.1
N$108  (via drill 0.5)
  Top 0.305: v30.16,42.55 28.3,40.68 23.22,40.68 22.52,39.98 5.42,39.98 v5.08,40.32
  Bottom 0.305: IC10.9 3.17,28.57 3.17,33.02 5.08,34.92 v5.08,40.32 | v30.16,42.55 30.8,42.55 33.02,44.77 33.02,46.67 33.34,46.99 45.09,46.99 45.72,46.35 45.72,40.64 | 45.72,40.64 45.72,37.78 46.99,36.51 RN3.3 | 113.1 58.42,41.91 53.98,41.91 X9.2.1 51.94,43.94 50.29,43.94 46.99,40.64 45.72,40.64
N$109  (via drill 0.5)
  Top 0.305: C18.1 115.57,7.62 116.2,7.62 116.84,8.26 116.84,9.53 115.57,10.79 108.9,10.79 | 108.9,10.79 94.3,10.79 91.76,8.26 84.45,8.26 R40.2 | 108.9,10.79 v108.9,10.86
  Bottom 0.305: IC11.13 110.49,16.51 110.49,13.97 108.9,12.38 v108.9,10.86
N$110  (via drill 0.5)
  Top 0.305: v44.45,21.91 44.83,21.91 45.09,22.16 51.82,22.16 53.02,20.95 67.94,20.95 68.54,20.36 77.03,20.36 77.75,21.08 79.5,21.08 X13.2.1
  Bottom 0.305: RN3.2 43.18,33.66 43.18,30.16 44.45,28.89 v44.45,21.91 | R40.1 80.01,10.16 80.01,21.59 X13.2.1
N$111  (via drill 0.5)
  Top 0.305: v104.14,12.38 103.12,11.43 93.98,11.43 | C17.1 93.98,11.43 | 93.98,11.43 92.08,9.53 90.17,9.53 89.53,10.16 80.01,10.16 R45.2
  Bottom 0.305: v104.14,12.38 IC9.4
N$112  (via drill 0.5)
  Top 0.305: v101.6,31.11 101.6,31.75 100.33,33.02 91.44,33.02 R43.2
  Bottom 0.305: v101.6,31.11 103.5,31.11 105.41,29.21 105.41,27.3 106.68,26.04 IC11.3
N$113  (via drill 0.5)
  Top 0.305: R43.1 v95.89,31.75
  Bottom 0.305: C15.1 92.71,24.13 91.44,25.4 91.44,28.89 92.71,30.16 R43.1 | IC8.9 95.89,31.11 v95.89,31.75
N$114  (via drill 0.5)
  Top 0.305: v93.66,8.26 92.39,6.99 55.24,6.99 R44.2 | v101.66,12.38 v94.61,12.38 | IC9.3 105.41,16.51 103.19,16.51 101.92,15.24 IC9.5
  Bottom 0.305: v93.66,8.26 94.61,9.21 v94.61,12.38 | v101.66,12.38 101.6,12.45 IC9.5
N$115  (via drill 0.5)
  Top 0.305: v48.9,2.22 49.53,1.59 89.53,1.59 90.17,2.22 | v90.49,4.45 90.49,2.54 90.17,2.22 | v108.27,32.38 110.81,29.84 v111.44,29.84 | v113.03,5.08 110.17,2.22 90.17,2.22
  Bottom 0.305: R44.1 50.8,8.26 48.39,5.84 48.39,2.73 v48.9,2.22 | v90.49,4.45 90.17,4.76 C16.1 | v108.27,32.38 107.95,32.38 106.68,33.66 IC8.3 | v111.44,29.84 112.08,29.84 113.03,28.89 113.03,23.18 112.71,22.86 112.71,20.95 113.03,20.64 v113.03,5.08
N$116  (via drill 0.5)
  Top 0.305: IC9.6 100.33,16.51 102.23,16.51 102.87,17.14 102.87,19.05 103.5,19.68 111.12,19.68 v113.67,22.23
  Bottom 0.305: v113.67,22.23 113.67,30.8 111.76,32.7 IC8.1

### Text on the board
bPlace: 60Hz
tNames: Sync. | Stunde | Minute | Wochentag | Tag | Monat | Jahr | V 1.1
